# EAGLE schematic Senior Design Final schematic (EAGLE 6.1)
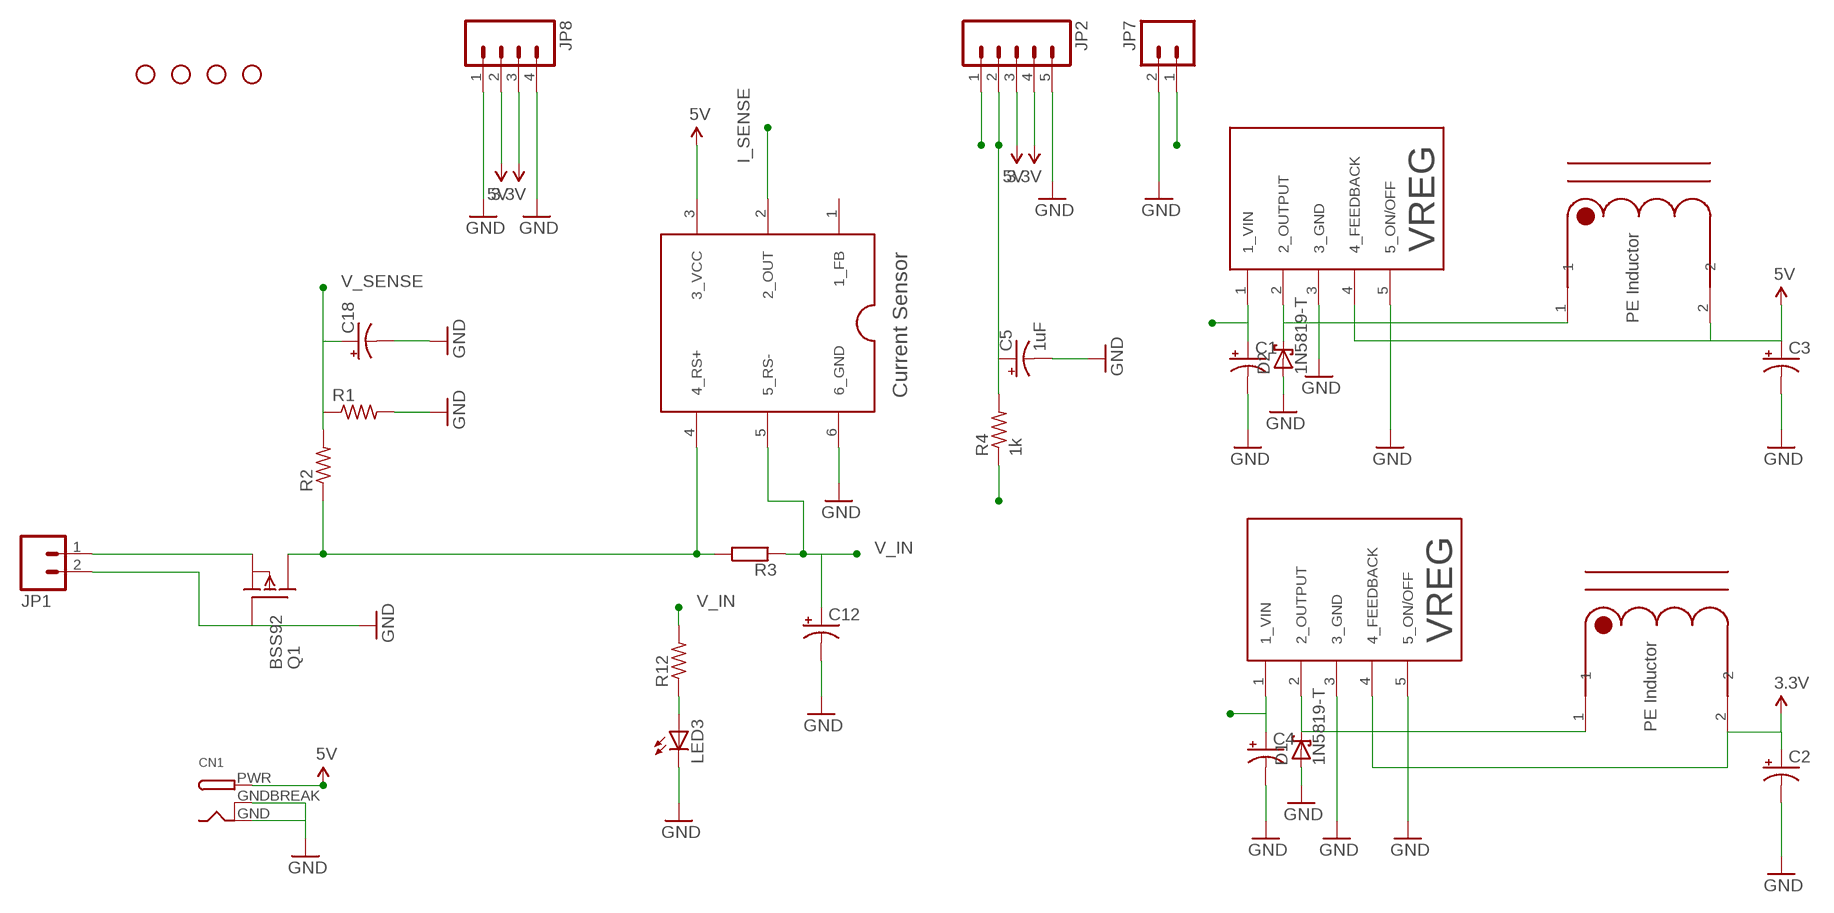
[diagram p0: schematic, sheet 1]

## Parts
C1  CAP_POLPTH1  [CPOL-RADIAL-100UF-25V]
C2  CAP_POLPTH1  [CPOL-RADIAL-100UF-25V]
C3  CAP_POLPTH1  [CPOL-RADIAL-100UF-25V]
C4  CAP_POLPTH1  [CPOL-RADIAL-100UF-25V]
C5  1uF  CAP_POLPTH1  [CPOL-RADIAL-100UF-25V]
C12  CAP_POLPTH1  [CPOL-RADIAL-100UF-25V]
C18  CAP_POLPTH1  [CPOL-RADIAL-100UF-25V]
CN1  DCBARRELPTH  [DCJACK_2MM_PTH]
D1  1N5819-T  [DO41-7.6]
D2  1N5819-T  [DO41-7.6]
JP1  M025MM  [SCREWTERMINAL-5MM-2]
JP2  M05LOCK  [1X05_LOCK]
JP3  STAND-OFF  [STAND-OFF]
JP4  STAND-OFF  [STAND-OFF]
JP5  STAND-OFF  [STAND-OFF]
JP6  STAND-OFF  [STAND-OFF]
JP7  M025MM  [SCREWTERMINAL-5MM-2]
JP8  M04LOCK  [1X04_LOCK]
LED3  LED5MM  [LED5MM]
Q1  BSS92  [TO92]
R1  R-US_0207/10  [0207/10]
R2  R-US_0207/10  [0207/10]
R3  SMK  [SMK]
R4  1k  R-US_0207/10  [0207/10]
R12  R-US_0207/10  [0207/10]
U$2  ISL28006  [ISL28006]
U$3  TL2575  [TL2575-05IKV]
U$4  PE-52627NL  [PE-52627NL]
U$6  TL2575  [TL2575-05IKV]
U$7  PE-52627NL  [PE-52627NL]

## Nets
3.3V: C2.1(+) JP2.4 JP8.3 U$3.4(4_FEEDBACK) U$4.2
5V: C3.1(+) CN1.PWR JP2.3 JP8.2 U$2.3(3_VCC) U$6.4(4_FEEDBACK) U$7.2
GND: C1.2(-) C2.2(-) C3.2(-) C4.2(-) C5.2(-) C12.2(-) C18.2(-) CN1.GND CN1.GNDBREAK D1.A D2.A JP1.2 JP2.5 JP7.2 JP8.1 JP8.4 LED3.K(C) Q1.1(G) R1.2 U$2.6(6_GND) U$3.3(3_GND) U$3.5(5_ON/OFF) U$6.3(3_GND) U$6.5(5_ON/OFF)
I_SENSE: R4.1 U$2.2(2_OUT)
N$1: JP1.1 Q1.3(S)
N$2: Q1.2(D) R2.1 R3.1 U$2.4(4_RS+)
N$4: LED3.A R12.1
N$5: D1.C U$3.2(2_OUTPUT) U$4.1
N$7: C5.1(+) JP2.2 R4.2
N$8: D2.C U$6.2(2_OUTPUT) U$7.1
V_IN: C1.1(+) C4.1(+) C12.1(+) JP7.1 R3.2 R12.2 U$2.5(5_RS-) U$3.1(1_VIN) U$6.1(1_VIN)
V_SENSE: C18.1(+) JP2.1 R1.1 R2.2
Unconnected: U$2.1(1_FB)

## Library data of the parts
C1-C5 C12 C18 = SparkFun-Passives:CAP_POL: Capacitor Polarized
CN1 = adafruit:DCBARREL: 2.0mm DC Barrel Jack DCJACK_2MM_PTH - Through Hole Jack (4UConnector: 05537)
D1 D2 = diode:1N581*: 1.0A SCHOTTKY BARRIER RECTIFIER
JP1 JP7 = SparkFun-Connectors:M02: Header 2
JP2 = SparkFun-Connectors:M05: Header 5 Standard 5-pin 0.1" header. Use with straight break away headers (SKU : PRT-00116), right angle break away headers (PRT-00553), swiss pins (PRT-00743), machine pins (PRT-00117), and female headers (PRT-00115). Molex polarized connector foot print use with SKU : PRT-08230 with associated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
JP3-JP6 = SparkFun-Electromechanical:STAND-OFF: #4 Stand Off
JP8 = SparkFun-Connectors:M04: Header 4 Standard 4-pin 0.1" header. Use with straight break away headers (SKU : PRT-00116), right angle break away headers (PRT-00553), swiss pins (PRT-00743), machine pins (PRT-00117), and female headers (PRT-00115). Molex polarized connector foot print use with SKU : PRT-08231 with associated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
LED3 = SparkFun-LED:LED: LEDs
Q1 = transistor-fet:BSS92: P-Channel Enhancement MOSFET -200V; -0,15A; 11Ohm
R1 R2 R4 R12 = rcl:R-US_: RESISTOR, American symbol
R3 = resistor-shunt:SMK: SMD SHUNT RESISTOR; OC_FARNELL: unknown; OC_NEWARK: unknown
U$2 = SD:ISL28006
U$3 U$6 = SD:TL2575
U$4 U$7 = SD:PE-52627NL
